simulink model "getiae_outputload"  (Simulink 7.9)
settings: Solver=ode23tb  StartTime=0.0  StopTime=400  RelTol=1e-6
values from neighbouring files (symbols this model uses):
  design = []    [sword.m]
libraries: simulink x2, cstextras x1

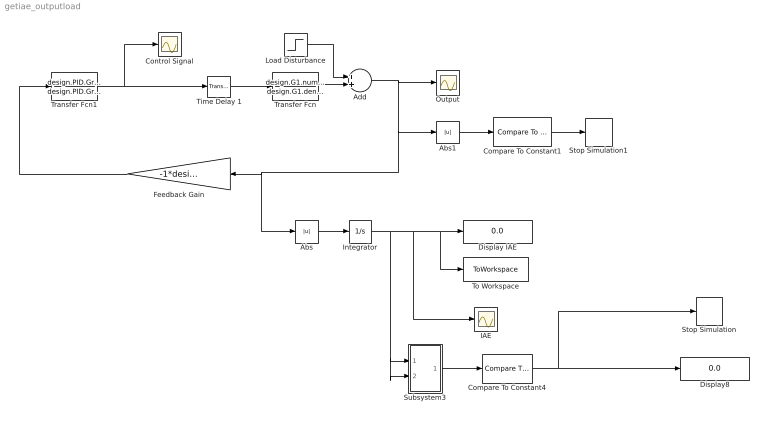
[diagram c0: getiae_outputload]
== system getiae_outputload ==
  Abs : Abs
  Abs1 : Abs
  Add : Sum
  Compare To Constant1 : simulink/Logic and Bit Operations/Compare To Constant  relop=>  const=5e12  OutDataTypeStr=boolean  ZeroCross=off
  Compare To Constant4 : simulink/Logic and Bit Operations/Compare To Constant  relop=<=  const=0.001  OutDataTypeStr=boolean  ZeroCross=off
  Control Signal : Scope
  Display IAE : Display
  Display8 : Display
  Feedback Gain : Gain  Gain=-1*design.sim.sgn
  IAE : Scope
  Integrator : Integrator
  Load Disturbance : Step  Time=0  SampleTime=0
  Output : Scope
  Stop Simulation : Stop
  Stop Simulation1 : Stop
  Subsystem3 : Subsystem
  Time Delay 1 : cstextras/Transport Delay (masked)  Tag=InputDelayBlock  Td=design.sim.L1  u0=0  bufsize=10000000
  To Workspace : ToWorkspace  VariableName=IAE_val  SampleTime=-1
  Transfer Fcn : TransferFcn  Numerator=design.G1.num{1}  Denominator=design.G1.den{1}
  Transfer Fcn1 : TransferFcn  Numerator=design.PID.Gr.num{1}  Denominator=design.PID.Gr.den{1}
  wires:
  Transfer Fcn1/1 -> Control Signal/1, Time Delay 1/1
  Time Delay 1/1 -> Transfer Fcn/1
  Feedback Gain/1 -> Transfer Fcn1/1
  Integrator/1 -> To Workspace/1, Display IAE/1, IAE/1, Subsystem3/1(In1), Subsystem3/2(In2)
  Subsystem3/1(Out1) -> Compare To Constant4/1
  Compare To Constant4/1 -> Display8/1, Stop Simulation/1
  Abs/1 -> Integrator/1
  Abs1/1 -> Compare To Constant1/1
  Compare To Constant1/1 -> Stop Simulation1/1
  Transfer Fcn/1 -> Add/2
  Load Disturbance/1 -> Add/1
  Add/1 -> Output/1, Abs1/1, Feedback Gain/1, Abs/1

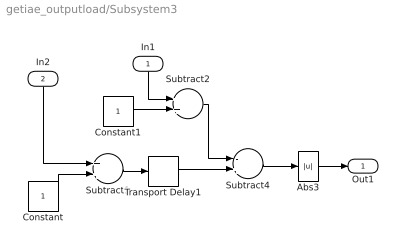
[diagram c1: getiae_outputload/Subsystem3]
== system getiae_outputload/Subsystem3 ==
  In1 : Inport
  In2 : Inport  Port=2
  Abs3 : Abs  ZeroCross=off
  Constant : Constant
  Constant1 : Constant
  Subtract1 : Sum
  Subtract2 : Sum
  Subtract4 : Sum  Inputs=-+
  Transport Delay1 : TransportDelay  DelayTime=50  BufferSize=100000
  Out1 : Outport
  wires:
  Abs3/1 -> Out1/1
  Subtract4/1 -> Abs3/1
  Transport Delay1/1 -> Subtract4/2
  Constant/1 -> Subtract1/2
  In2/1 -> Subtract1/1
  Subtract1/1 -> Transport Delay1/1
  Constant1/1 -> Subtract2/2
  Subtract2/1 -> Subtract4/1
  In1/1 -> Subtract2/1
